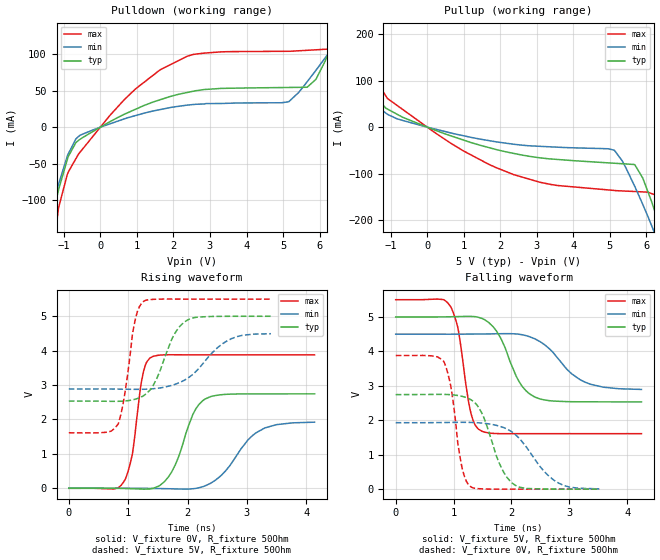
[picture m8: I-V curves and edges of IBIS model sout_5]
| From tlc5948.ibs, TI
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|   sout_5 Model
[Model]   sout_5
Model_type   Output
Polarity   Non-Inverting
Vmeas = 2.5
Vref = 2.5
Cref = 15pF
Rref = 50
|   typ   min   max
|   (nom PVT)   (fast PVT)   (slow PVT)
|C_comp from frequency sweep method (F=8.25MHz)
|C_comp   1.758e-12   1.750e-12   1.791e-12
|ON state : BUFFER OUTPUT TURNED HIGH
|C_comp   1.758e-12   1.750e-12   1.791e-12
|OFF state: BUFFER OUTPUT TURNED LOW
|C_comp   2.045e-12   1.993e-12   2.309e-12
|C_comp from LC tank measurement(L=1nH)
|Resonant Frequency(Hz)   4.650e+09   4.760e+09   4.280e+09
C_comp   1.173e-12   1.119e-12   1.384e-12
|ON state : BUFFER OUTPUT TURNED HIGH
|Resonant Frequency(Hz)   4.650e+09   4.760e+09   4.280e+09
|C_comp   1.173e-12   1.119e-12   1.384e-12
|OFF state: BUFFER OUTPUT TURNED LOW
|Resonant Frequency(Hz)   4.440e+09   4.560e+09   4.140e+09
|C_comp   1.286e-12   1.219e-12   1.479e-12
| Where nom  PVT is Nominal Process, 5V, 90C
|   Fast PVT is Strong Process,  5.5V, -40C
|   Slow PVT is Weak Process,   4.5V, 150C
[Voltage Range]   5   4.5   5.5
|Ambient Temperature   25   85   -40
|Junction Temperature
[Temperature Range]   90   150   -40
[Pullup Reference]   5   4.5   5.5
[Pulldown Reference]   0   0   0
[Power Clamp Reference]   5   4.5   5.5
[GND Clamp Reference]   0   0   0
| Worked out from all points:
|   slope of the pulldown table from 0 to 0.75 V, typ, clamps not added: 37.9 ohm
|   slope of the pullup table from 0 to 0.75 V, typ, clamps not added: 35 ohm
|   falling waveform, V_fixture 5V, R_fixture 50Ohm: 20-80 % time 396ps typ, 570ps min, 206ps max; typ from 5 V to 2.54 V
|   rising waveform, V_fixture 0V, R_fixture 50Ohm: 20-80 % time 350ps typ, 526ps min, 183ps max; typ from 0 V to 2.75 V
|   rising waveform, V_fixture 5V, R_fixture 50Ohm: 20-80 % time 356ps typ, 558ps min, 192ps max; typ from 2.54 V to 5 V
|   falling waveform, V_fixture 0V, R_fixture 50Ohm: 20-80 % time 356ps typ, 547ps min, 191ps max; typ from 2.75 V to 0 V
[Pulldown]
|   Voltage   I(typ)   I(min)   I(max)
-5V       -1.068A    -850.4mA   -1.617A
-2.115V   -320.5mA   -254.8mA   -541.4mA
-1.373V   -136.9mA   -115mA     -201.7mA
-670mV    -21.23mA   -16.19mA   -43.23mA
968mV     24.65mA    15.96mA    52.69mA
2.376V    47.53mA    30.2mA     97.26mA
5.157V    54.43mA    34.86mA    104.1mA
5.9V      65.54mA    77.93mA    106.1mA
6.418V    119.6mA    113mA      107.7mA
6.556V    134.9mA    122.3mA    127.8mA
6.835V    166mA      141.1mA    207.1mA
10V       485.2mA    347.8mA    890.7mA
[Pullup]
|   Voltage   I(typ)   I(min)   I(max)
-5V       430.2mA    280.3mA    839.4mA
-4.004V   339.2mA    217.9mA    718mA
-2.728V   208.6mA    134.5mA    483.2mA
-2.332V   166.2mA    108.2mA    387.3mA
-1.14V    41.08mA    30.63mA    67.92mA
968mV     -27.14mA   -18.14mA   -50.18mA
3.08V     -65.98mA   -41.27mA   -118.6mA
5.117V    -77.69mA   -49.64mA   -136.3mA
5.685V    -81.4mA    -128.4mA   -138.6mA
6.303V    -198mA     -243.3mA   -147.7mA
6.6V      -269.6mA   -301.1mA   -216.8mA
10V       -1.153A    -1.008A    -1.611A
[Ramp]
R_load = 50
|   typ   min   max
dV/dt_r   1.64723/3.47953e-10   1.15712/5.27212e-10   2.32784/1.82223e-10
dV/dt_f   1.47932/3.94388e-10   0.967312/5.6894e-10   2.33259/2.05872e-10
[Falling Waveform]
V_fixture = 5V
V_fixture_min = 4.5V
V_fixture_max = 5.5V
R_fixture = 50Ohm
|   Time   V(typ)   V(min)   V(max)
0s        5V         4.5V       5.5V
950ps     5.005V     4.499V     5.297V
1.07ns    5.01V      4.5V       4.719V
1.3ns     5.016V     4.502V     2.205V
1.49ns    4.957V     4.505V     1.681V
1.74ns    4.594V     4.511V     1.614V
2.115ns   3.17V      4.501V     1.612V
2.395ns   2.681V     4.37V      1.612V
3.265ns   2.536V     3.111V     1.612V
4.245ns   2.535V     2.895V     1.612V
[Rising Waveform]
V_fixture = 0V
V_fixture_min = 0V
V_fixture_max = 0V
R_fixture = 50Ohm
|   Time   V(typ)   V(min)   V(max)
0s        8.672nV    29.37nV    1.176nV
935ps     -6.485mV   755.8uV    214.5mV
1.07ns    -13.54mV   383.6uV    988.4mV
1.255ns   -25.98mV   -2.093mV   3.369V
1.365ns   -20.17mV   -4.411mV   3.785V
1.73ns    465.9mV    -15.58mV   3.882V
2.09ns    2.147V     -14.03mV   3.88V
2.29ns    2.589V     66.72mV    3.88V
3.15ns    2.744V     1.609V     3.88V
4.14ns    2.745V     1.922V     3.88V
[Rising Waveform]
V_fixture = 5V
V_fixture_min = 4.5V
V_fixture_max = 5.5V
R_fixture = 50Ohm
|   Time   V(typ)   V(min)   V(max)
0s        2.535V     2.887V     1.613V
830ps     2.528V     2.882V     1.864V
940ps     2.538V     2.88V      2.721V
1.115ns   2.588V     2.876V     4.869V
1.26ns    2.692V     2.878V     5.433V
1.425ns   3.002V     2.894V     5.492V
1.75ns    4.387V     2.999V     5.5V
1.96ns    4.847V     3.155V     5.5V
2.67ns    4.999V     4.289V     5.5V
3.405ns   5V         4.493V     5.5V
[Falling Waveform]
V_fixture = 0V
V_fixture_min = 0V
V_fixture_max = 0V
R_fixture = 50Ohm
|   Time   V(typ)   V(min)   V(max)
0s        2.745V     1.929V     3.879V
830ps     2.751V     1.935V     3.71V
950ps     2.742V     1.937V     3.004V
1.145ns   2.695V     1.94V      630.2mV
1.31ns    2.584V     1.937V     53.46mV
1.515ns   2.109V     1.915V     6.626mV
1.855ns   523.4mV    1.793V     -451uV
2.06ns    117mV      1.595V     -134.1uV
2.73ns    1.119mV    264.1mV    26.5uV
3.515ns   68.42uV    7.904mV    16.21uV
